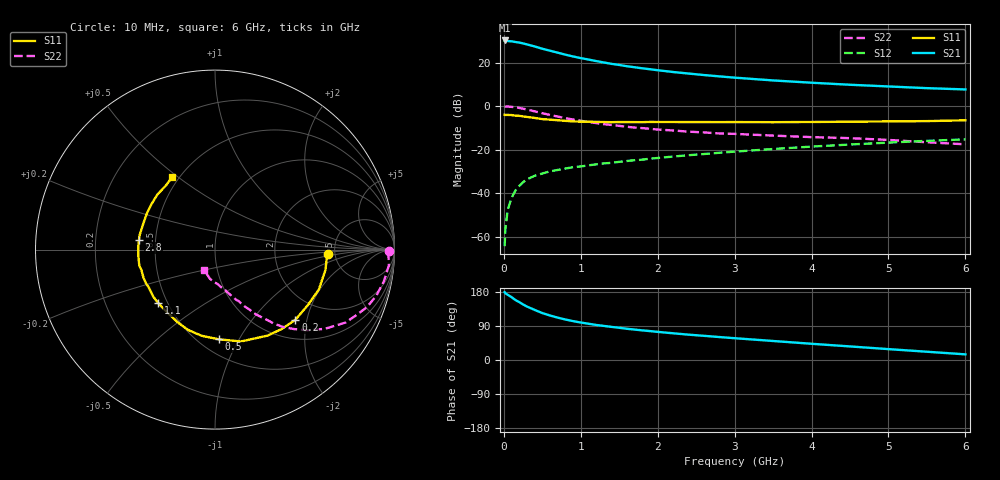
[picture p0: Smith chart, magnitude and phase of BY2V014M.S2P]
! SIEMENS Small Signal Semiconductors
! BFY420
! Si NPN RF SIEGET Grounded Emitter Transistor in MICRO-X
! VCE = 2 V  IC = 14 mA
! Common Emitter S-Parameters:  October  1996
# GHz  S  MA  R  50
!  f  S11  S21  S12  S22
! GHz  MAG  ANG  MAG  ANG  MAG  ANG  MAG  ANG
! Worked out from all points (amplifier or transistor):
!   36 points, 10 MHz to 6 GHz, reference 50 ohm
!   highest |S21| = 30.1 dB at 10 MHz (marker M1)
!   |S21| within 3 dB of that: start of sweep to 423.5 MHz
!   unconditionally stable (mu >= 1): 2.23 GHz to end of sweep
!   at 250 MHz: K = 0.26, MSG = 31.9 dB, |S12| = -35.0 dB
!   at 1.4 GHz: K = 0.85, MSG = 22.8 dB, |S12| = -26.1 dB
!   at 6 GHz: K = 1.09, MAG = 9.7 dB, |S12| = -15.3 dB
!   S11 on the Smith chart (normalised r, x): 10 MHz: 4.34, -0.38; 200 MHz: 1.41, -1.71; 500 MHz: 0.62, -0.83; 1.1 GHz: 0.45, -0.33; 2.8 GHz: 0.40, +0.05; 6 GHz: 0.46, +0.48
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0.01  0.6276 -2.4  32.16 178.9  0.0006 96.6  0.9717 -0.6
0.02  0.6244 -4.7  31.9 176.2  0.0015 98.3  0.967 -1.8
0.1  0.6198 -21.1  30.71 165.9  0.0077 82.5  0.957 -10.8
0.15  0.6028 -30.8  29.64 158.3  0.0114 76.2  0.9344 -16.0
0.2  0.5946 -41.1  28.75 152.8  0.0145 73.7  0.9055 -20.7
0.25  0.5777 -50.0  27.49 146.5  0.0177 66.7  0.8662 -25.1
0.3  0.5619 -58.5  26.1 141.1  0.0206 66.4  0.8331 -29.2
0.4  0.5318 -74.3  23.43 132.3  0.0249 61.8  0.7544 -35.8
0.5  0.5001 -87.6  20.76 123.8  0.0281 58.9  0.6841 -41.1
0.6  0.4859 -98.9  18.69 117.5  0.0315 56.3  0.6239 -45.2
0.7  0.4719 -108.6  16.85 111.8  0.0339 54.7  0.5722 -48.8
0.8  0.4559 -116.8  15.16 106.9  0.0366 53.0  0.5262 -51.5
0.9  0.4432 -124.0  13.77 102.6  0.0392 52.5  0.4888 -53.4
1.1  0.4342 -136.8  11.71 95.7  0.0432 52.5  0.43 -57.5
1.3  0.4279 -146.3  10.03 89.9  0.048 52.3  0.384 -60.2
1.6  0.4279 -158.7  8.219 82.4  0.0545 52.0  0.3334 -64.1
2.2  0.4286 -175.0  6.051 70.5  0.069 51.1  0.2742 -70.3
2.8  0.4269 172.7  4.806 60.6  0.0841 49.0  0.2343 -75.7
3.5  0.4251 159.8  3.875 50.2  0.1027 45.1  0.209 -81.5
4.5  0.4354 144.3  3.082 35.8  0.1303 37.9  0.1826 -90.7
5.5  0.45 127.4  2.576 21.8  0.1583 29.3  0.1469 -106.9
6  0.4699 120.3  2.406 14.9  0.1713 24.5  0.1317 -118.6
